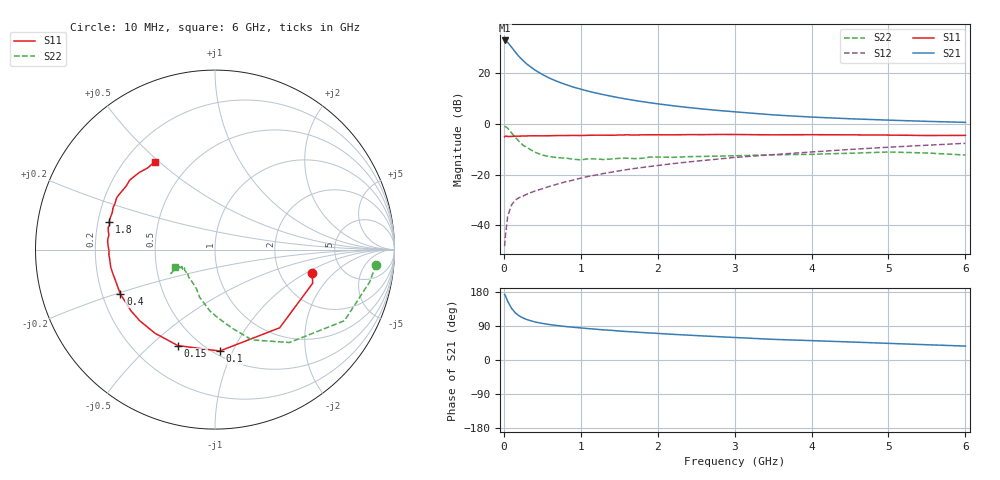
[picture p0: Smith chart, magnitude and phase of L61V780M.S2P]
!  INFINEON TECHNOLOGIES Small Signal Semiconductors
! BFR380L3 , Si-NPN RF-Transistor in TSLP-3-1
!  Vce=1.75 V,  Ic=80 mA
! Common Emitter S-Parameters:  07. March 2005
#  GHz  S  MA  R  50
! f  S11  S21  S12  S22
! GHz  Mag  Ang  Mag  Ang  Mag  Ang  Mag  Ang
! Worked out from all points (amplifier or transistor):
!   36 points, 10 MHz to 6 GHz, reference 50 ohm
!   highest |S21| = 32.9 dB at 10 MHz (marker M1)
!   |S21| within 3 dB of that: start of sweep to 109.3 MHz
!   unconditionally stable (mu >= 1): 994.3 MHz to 5.632 GHz
!   at 250 MHz: K = 0.56, MSG = 26.7 dB, |S12| = -28.5 dB
!   at 1.4 GHz: K = 1.04, MAG = 13.7 dB, |S12| = -19.0 dB
!   at 6 GHz: K = 0.99, MSG = 4.1 dB, |S12| = -7.7 dB
!   S11 on the Smith chart (normalised r, x): 10 MHz: 3.03, -1.15; 100 MHz: 0.54, -0.89; 150 MHz: 0.39, -0.61; 400 MHz: 0.28, -0.21; 1.8 GHz: 0.25, +0.12; 6 GHz: 0.32, +0.48
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0.01  0.5574 -13.6  43.96 173.2  0.0039 67.4  0.9006 -5.4
0.02  0.5756 -19.0  43.49 169.9  0.0062 80.6  0.8806 -11.8
0.05  0.5653 -50.4  40.18 154.9  0.0151 68.7  0.8228 -28.8
0.1  0.5657 -87.3  32.46 136.5  0.0253 58.0  0.6633 -51.3
0.15  0.5734 -111.1  25.86 124.2  0.0317 52.3  0.5434 -67.8
0.2  0.5736 -125.7  21.04 116.4  0.0353 50.6  0.4495 -77.5
0.25  0.577 -136.5  17.64 110.8  0.0378 49.7  0.3788 -87.9
0.3  0.5792 -143.9  15.02 106.6  0.0413 50.6  0.3421 -94.9
0.4  0.5825 -154.9  11.61 100.6  0.0474 52.7  0.279 -107.9
0.5  0.5804 -162.0  9.421 96.6  0.0528 55.1  0.2423 -115.1
0.6  0.5848 -166.9  7.871 93.4  0.0592 57.7  0.2264 -121.9
0.7  0.5891 -170.4  6.804 90.8  0.0654 59.8  0.2158 -128.5
0.9  0.592 -177.5  5.317 86.5  0.078 62.2  0.2019 -138.4
1.1  0.5957 178.2  4.399 82.8  0.0922 64.2  0.205 -142.0
1.4  0.5964 172.3  3.491 78.3  0.1119 65.4  0.2031 -147.0
1.8  0.6081 165.4  2.742 72.5  0.1387 66.2  0.21 -152.0
2.2  0.6086 160.1  2.274 67.7  0.1649 66.2  0.2191 -152.6
2.8  0.6191 152.4  1.832 61.4  0.2037 65.9  0.2317 -156.2
3.5  0.6083 144.4  1.504 54.5  0.2476 63.6  0.2461 -154.0
4.5  0.6077 138.0  1.261 47.6  0.3134 61.4  0.2641 -152.6
5.5  0.5898 129.6  1.121 40.3  0.38 57.2  0.2669 -152.7
6  0.5932 124.5  1.07 36.7  0.414 54.8  0.2432 -156.5
